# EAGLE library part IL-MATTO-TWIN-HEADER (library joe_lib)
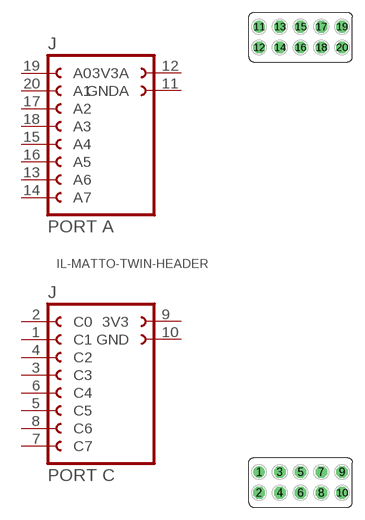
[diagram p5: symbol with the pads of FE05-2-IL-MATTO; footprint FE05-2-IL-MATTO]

Designator prefix J

## IL-MATTO-TWIN-HEADER  [FE05-2-IL-MATTO]
1  C1
2  C0
3  C3
4  C2
5  C5
6  C4
7  C7
8  C6
9  3V3  pwr
10  GND  pwr
11  GNDA  pwr
12  3V3A  pwr
13  A6
14  A7
15  A4
16  A5
17  A2
18  A3
19  A0
20  A1

## Footprint FE05-2-IL-MATTO (pad centres in mm)
FEMALE HEADER
drill 0.914: 1 -5.08,1.27; 11 -5.08,55.88
drill 0.914 octagon: 2 -5.08,-1.27; 3 -2.54,1.27; 4 -2.54,-1.27; 5 0,1.27; 6 0,-1.27; 7 2.54,1.27; 8 2.54,-1.27; 9 5.08,1.27; 10 5.08,-1.27; 12 -5.08,53.34; 13 -2.54,55.88; 14 -2.54,53.34; 15 0,55.88; 16 0,53.34; 17 2.54,55.88; 18 2.54,53.34; 19 5.08,55.88; 20 5.08,53.34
